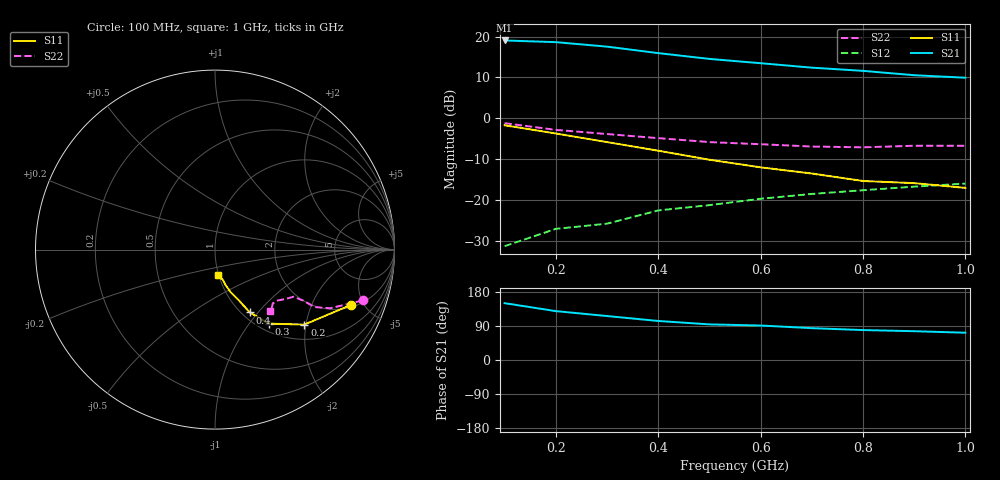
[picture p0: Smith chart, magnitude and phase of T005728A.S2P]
!AT-00572
!S-PARAMETERS at Vce=8V  Ic=5mA.  LAST UPDATED 07-21-92
# ghz s ma r 50
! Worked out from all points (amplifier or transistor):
!   10 points, 100 MHz to 1 GHz, reference 50 ohm
!   highest |S21| = 19.1 dB at 100 MHz (marker M1)
!   |S21| within 3 dB of that: start of sweep to 393.6 MHz
!   unconditionally stable (mu >= 1): 603.3 MHz to end of sweep
!   at 200 MHz: K = 0.57, MSG = 22.9 dB, |S12| = -27.1 dB
!   at 600 MHz: K = 1.00, MSG = 16.6 dB, |S12| = -19.7 dB
!   at 1 GHz: K = 1.03, MAG = 11.9 dB, |S12| = -16.0 dB
!   S11 on the Smith chart (normalised r, x): 100 MHz: 2.16, -4.05; 200 MHz: 1.35, -1.96; 300 MHz: 1.12, -1.25; 400 MHz: 1.09, -0.91; 1 GHz: 0.99, -0.28
0.1  0.82 -22.0  8.99 150.0  0.027 75.0  0.87 -19.0
0.2  0.65 -40.0  8.57 129.0  0.044 72.0  0.72 -27.0
0.3  0.51 -54.0  7.55 116.0  0.051 69.0  0.64 -30.0
0.4  0.4 -61.0  6.29 103.0  0.074 66.0  0.57 -30.0
0.5  0.31 -65.0  5.34 94.0  0.086 65.0  0.51 -31.0
0.6  0.25 -70.0  4.73 91.0  0.103 67.0  0.48 -35.0
0.7  0.21 -73.0  4.17 84.0  0.118 65.0  0.45 -39.0
0.8  0.17 -76.0  3.81 79.0  0.131 64.0  0.44 -43.0
0.9  0.16 -81.0  3.37 76.0  0.145 65.0  0.46 -47.0
1  0.14 -83.0  3.14 72.0  0.158 64.0  0.46 -48.0
